| IBIS file stm32g030_031_041_tssop20.ibs
[IBIS ver] 4.2
[File name] stm32g030_031_041_tssop20.ibs
[File Rev] rev1.1
[Date]  15-05-2022
[Source] Data Created at STMicroelectronics
[Notes]  File originated from ELDO simulations.
[Disclaimer]  This information is for modeling purpose only and is
   not guaranted. The information is subject to change without
   notice.
[Copyright] Copyright 2022 STMicroelectronics Inc.
|   Component stm32g030_031_041_tssop20
[Component] stm32g030_031_041_tssop20
[Manufacturer] STMicroelectronics
[Package]
| variable   typ   min   max
R_pkg   0.0   0.0   0.0
L_pkg   0.0H   0.0H   0.0H
C_pkg   0.0F   0.0F   0.0F
[Pin]   signal_name   model_name  R_pin L_pin C_pin
1 PB8 io6_i2c_ft
2 PC14-OSCI32_IN io6_i2c_ft
3 PC15-OSC32_OUT io8prog2m25m50m120m_sudq_ft
4 VDD POWER
5 VSS GND
6 PF2-NRST io6reset
7 PA0 io6_ft
8 PA1 io6_ft
9 PA2 io6_ft
10 PA3 io6_ft
11 PA4 io6_ft
12 PA5 io6_ft
13 PA6 io6_ft
14 PA7 io6_ft
15 PB0 io6_ft
16 PA11 io6_i2c_ft
17 PA12 io6_i2c_ft
18 PA13 io6_ft
19 PA15 io6_ft
20 PB6 io6_i2c_ft
[Model Selector] io8prog2m25m50m120m_sudq_ft
iols8p_sudq_ft_pd_lv  "IO low speed, PD=40kOhm - 1P8V"
iols8p_sudq_ft_pu_lv  "IO low speed, PU=40kOhm - 1P8V"
iols8p_sudq_ft_lv  "IO low speed - 1P8V"
iols8p_sudq_ft_pd  "IO low speed, PD=40kOhm - 3P3V"
iols8p_sudq_ft_pu  "IO low speed, PU=40kOhm - 3P3V"
iols8p_sudq_ft  "IO low speed - 3P3V"
iofs8p_sudq_ft_pd_lv  "IO full speed, PD=40kOhm - 1P8V"
iofs8p_sudq_ft_pu_lv  "IO full speed, PU=40kOhm - 1P8V"
iofs8p_sudq_ft_lv  "IO full speed - 1P8V"
iofs8p_sudq_ft_pd  "IO full speed, PD=40kOhm - 3P3V"
iofs8p_sudq_ft_pu  "IO full speed, PU=40kOhm - 3P3V"
iofs8p_sudq_ft  "IO full speed - 3P3V"
ioms8p_sudq_ft_pd_lv  "IO medium speed, PD=40kOhm - 1P8V"
ioms8p_sudq_ft_pu_lv  "IO medium speed, PU=40kOhm - 1P8V"
ioms8p_sudq_ft_lv  "IO medium speed - 1P8V"
ioms8p_sudq_ft_pd  "IO medium speed, PD=40kOhm - 3P3V"
ioms8p_sudq_ft_pu  "IO medium speed, PU=40kOhm - 3P3V"
ioms8p_sudq_ft  "IO medium speed - 3P3V"
iohs8p_sudq_ft_pd_lv  "IO high speed, PD=40kOhm - 1P8V"
iohs8p_sudq_ft_pu_lv  "IO high speed, PU=40kOhm - 1P8V"
iohs8p_sudq_ft_lv  "IO high speed - 1P8V"
iohs8p_sudq_ft_pd  "IO high speed, PD=40kOhm - 3P3V"
iohs8p_sudq_ft_pu  "IO high speed, PU=40kOhm - 3P3V"
iohs8p_sudq_ft  "IO high speed - 3P3V"
[Model Selector] io6_ft
io6_ft_1v8_highspeed_pd  "GPIO-1.8V range - high speed - pull down"
io6_ft_1v8_fastspeed_pd  "GPIO-1.8V range - fast speed - pull down"
io6_ft_1v8_mediumspeed_pd  "GPIO-1.8V range - medium speed - pull down"
io6_ft_1v8_lowspeed_pd  "GPIO-1.8V range - low speed - pull down"
io6_ft_1v8_highspeed_pu  "GPIO-1.8V range - high speed - pull up"
io6_ft_1v8_fastspeed_pu  "GPIO-1.8V range - fast speed - pull up"
io6_ft_1v8_mediumspeed_pu  "GPIO-1.8V range - medium speed - pull up"
io6_ft_1v8_lowspeed_pu  "GPIO-1.8V range - low speed - pull up"
io6_ft_1v8_highspeed  "GPIO-1.8V range - high speed"
io6_ft_1v8_fastspeed  "GPIO-1.8V range - fast speed"
io6_ft_1v8_mediumspeed  "GPIO-1.8V range - medium speed"
io6_ft_1v8_lowspeed  "GPIO-1.8V range - low speed"
io6_ft_3v3_highspeed_pd  "GPIO-3.3V range - high speed - pull down"
io6_ft_3v3_fastspeed_pd  "GPIO-3.3V range - fast speed - pull down"
io6_ft_3v3_mediumspeed_pd  "GPIO-3.3V range - medium speed - pull down"
io6_ft_3v3_lowspeed_pd  "GPIO-3.3V range - low speed - pull down"
io6_ft_3v3_highspeed_pu  "GPIO-3.3V range - high speed - pull up"
io6_ft_3v3_fastspeed_pu  "GPIO-3.3V range - fast speed - pull up"
io6_ft_3v3_mediumspeed_pu  "GPIO-3.3V range - medium speed - pull up"
io6_ft_3v3_lowspeed_pu  "GPIO-3.3V range - low speed - pull up"
io6_ft_3v3_highspeed  "GPIO-3.3V range - high speed"
io6_ft_3v3_fastspeed  "GPIO-3.3V range - fast speed"
io6_ft_3v3_mediumspeed  "GPIO-3.3V range - medium speed"
io6_ft_3v3_lowspeed  "GPIO-3.3V range - low speed"
[Model Selector] io6_i2c_ft
io6_ft_1v8_highspeed_pd  "GPIO-1.8V range - high speed - pull down"
io6_ft_1v8_fastspeed_pd  "GPIO-1.8V range - fast speed - pull down"
io6_ft_1v8_mediumspeed_pd  "GPIO-1.8V range - medium speed - pull down"
io6_ft_1v8_lowspeed_pd  "GPIO-1.8V range - low speed - pull down"
io6_ft_1v8_highspeed_pu  "GPIO-1.8V range - high speed - pull up"
io6_ft_1v8_fastspeed_pu  "GPIO-1.8V range - fast speed - pull up"
io6_ft_1v8_mediumspeed_pu  "GPIO-1.8V range - medium speed - pull up"
io6_ft_1v8_lowspeed_pu  "GPIO-1.8V range - low speed - pull up"
io6_ft_1v8_highspeed  "GPIO-1.8V range - high speed"
io6_ft_1v8_fastspeed  "GPIO-1.8V range - fast speed"
io6_ft_1v8_mediumspeed  "GPIO-1.8V range - medium speed"
io6_ft_1v8_lowspeed  "GPIO-1.8V range - low speed"
io6_ft_3v3_highspeed_pd  "GPIO-3.3V range - high speed - pull down"
io6_ft_3v3_fastspeed_pd  "GPIO-3.3V range - fast speed - pull down"
io6_ft_3v3_mediumspeed_pd  "GPIO-3.3V range - medium speed - pull down"
io6_ft_3v3_lowspeed_pd  "GPIO-3.3V range - low speed - pull down"
io6_ft_3v3_highspeed_pu  "GPIO-3.3V range - high speed - pull up"
io6_ft_3v3_fastspeed_pu  "GPIO-3.3V range - fast speed - pull up"
io6_ft_3v3_mediumspeed_pu  "GPIO-3.3V range - medium speed - pull up"
io6_ft_3v3_lowspeed_pu  "GPIO-3.3V range - low speed - pull up"
io6_ft_3v3_highspeed  "GPIO-3.3V range - high speed"
io6_ft_3v3_fastspeed  "GPIO-3.3V range - fast speed"
io6_ft_3v3_mediumspeed  "GPIO-3.3V range - medium speed"
io6_ft_3v3_lowspeed  "GPIO-3.3V range - low speed"
io6_ft_1v8_highi2c_pd   "GPIO-1.8V range - high   speed i2c mode - pd"
io6_ft_1v8_fasti2c_pd   "GPIO-1.8V range - fast   speed i2c mode - pd"
io6_ft_1v8_mediumi2c_pd  "GPIO-1.8V range - medium speed i2c mode - pd"
io6_ft_1v8_lowi2c_pd   "GPIO-1.8V range - low   speed i2c mode - pd"
io6_ft_1v8_highi2c_pu   "GPIO-1.8V range - high   speed i2c mode - pu"
io6_ft_1v8_fasti2c_pu   "GPIO-1.8V range - fast   speed i2c mode - pu"
io6_ft_1v8_mediumi2c_pu  "GPIO-1.8V range - medium speed i2c mode - pu"
io6_ft_1v8_lowi2c_pu   "GPIO-1.8V range - low   speed i2c mode - pu"
io6_ft_1v8_highi2c   "GPIO-1.8V range - high   speed i2c mode"
io6_ft_1v8_fasti2c   "GPIO-1.8V range - fast   speed i2c mode"
io6_ft_1v8_mediumi2c   "GPIO-1.8V range - medium speed i2c mode"
io6_ft_1v8_lowi2c   "GPIO-1.8V range - low   speed i2c mode"
io6_ft_3v3_highi2c_pd   "GPIO-3.3V range - high   speed i2c mode - pd"
io6_ft_3v3_fasti2c_pd   "GPIO-3.3V range - fast   speed i2c mode - pd"
io6_ft_3v3_mediumi2c_pd  "GPIO-3.3V range - medium speed i2c mode - pd"
io6_ft_3v3_lowi2c_pd   "GPIO-3.3V range - low   speed i2c mode - pd"
io6_ft_3v3_highi2c_pu   "GPIO-3.3V range - high   speed i2c mode - pu"
io6_ft_3v3_fasti2c_pu   "GPIO-3.3V range - fast   speed i2c mode - pu"
io6_ft_3v3_mediumi2c_pu  "GPIO-3.3V range - medium speed i2c mode - pu"
io6_ft_3v3_lowi2c_pu   "GPIO-3.3V range - low   speed i2c mode - pu"
io6_ft_3v3_highi2c   "GPIO-3.3V range - high   speed i2c mode"
io6_ft_3v3_fasti2c   "GPIO-3.3V range - fast   speed i2c mode"
io6_ft_3v3_mediumi2c   "GPIO-3.3V range - medium speed i2c mode"
io6_ft_3v3_lowi2c   "GPIO-3.3V range - low   speed i2c mode"
io6_i2c_ft_1v8_pd  "GPIO-1.8V I2C fm+ - pd"
io6_i2c_ft_3v3_pd  "GPIO-3.3V I2C fm+ - pd"
io6_i2c_ft_1v8_pu  "GPIO-1.8V I2C fm+ - pu"
io6_i2c_ft_3v3_pu  "GPIO-3.3V I2C fm+ - pu"
io6_i2c_ft_1v8   "GPIO-1.8V I2C fm+"
io6_i2c_ft_3v3   "GPIO-3.3V I2C fm+"
[Model Selector] io6reset
io6_ft_1v8_highspeed_pd  "GPIO-1.8V range - high speed - pull down"
io6_ft_1v8_fastspeed_pd  "GPIO-1.8V range - fast speed - pull down"
io6_ft_1v8_mediumspeed_pd  "GPIO-1.8V range - medium speed - pull down"
io6_ft_1v8_lowspeed_pd  "GPIO-1.8V range - low speed - pull down"
io6_ft_1v8_highspeed_pu  "GPIO-1.8V range - high speed - pull up"
io6_ft_1v8_fastspeed_pu  "GPIO-1.8V range - fast speed - pull up"
io6_ft_1v8_mediumspeed_pu  "GPIO-1.8V range - medium speed - pull up"
io6_ft_1v8_lowspeed_pu  "GPIO-1.8V range - low speed - pull up"
io6_ft_1v8_highspeed  "GPIO-1.8V range - high speed"
io6_ft_1v8_fastspeed  "GPIO-1.8V range - fast speed"
io6_ft_1v8_mediumspeed  "GPIO-1.8V range - medium speed"
io6_ft_1v8_lowspeed  "GPIO-1.8V range - low speed"
io6_ft_3v3_highspeed_pd  "GPIO-3.3V range - high speed - pull down"
io6_ft_3v3_fastspeed_pd  "GPIO-3.3V range - fast speed - pull down"
io6_ft_3v3_mediumspeed_pd  "GPIO-3.3V range - medium speed - pull down"
io6_ft_3v3_lowspeed_pd  "GPIO-3.3V range - low speed - pull down"
io6_ft_3v3_highspeed_pu  "GPIO-3.3V range - high speed - pull up"
io6_ft_3v3_fastspeed_pu  "GPIO-3.3V range - fast speed - pull up"
io6_ft_3v3_mediumspeed_pu  "GPIO-3.3V range - medium speed - pull up"
io6_ft_3v3_lowspeed_pu  "GPIO-3.3V range - low speed - pull up"
io6_ft_3v3_highspeed  "GPIO-3.3V range - high speed"
io6_ft_3v3_fastspeed  "GPIO-3.3V range - fast speed"
io6_ft_3v3_mediumspeed  "GPIO-3.3V range - medium speed"
io6_ft_3v3_lowspeed  "GPIO-3.3V range - low speed"
ioreset_1v2_pu  "RESET 1.2V range with PU"
ioreset_1v2  "RESET 1.2V range"
ioreset_1v8_pu  "RESET 1.8V range with PU"
ioreset_1v8  "RESET 1.8V range"
ioreset_3v3_pu  "RESET 3.3V range with PU"
ioreset_3v3  "RESET 3.3V range"
| Models and submodels in the file (84): iols8p_sudq_ft_pd_lv (I/O), iols8p_sudq_ft_pu_lv (I/O), iols8p_sudq_ft_lv (I/O), iols8p_sudq_ft_pd (I/O), iols8p_sudq_ft_pu (I/O), iols8p_sudq_ft (I/O), iofs8p_sudq_ft_pd_lv (I/O), iofs8p_sudq_ft_pu_lv (I/O), iofs8p_sudq_ft_lv (I/O), iofs8p_sudq_ft_pd (I/O), iofs8p_sudq_ft_pu (I/O), iofs8p_sudq_ft (I/O), ioms8p_sudq_ft_pd_lv (I/O), ioms8p_sudq_ft_pu_lv (I/O), ioms8p_sudq_ft_lv (I/O), ioms8p_sudq_ft_pd (I/O), ioms8p_sudq_ft_pu (I/O), ioms8p_sudq_ft (I/O), iohs8p_sudq_ft_pd_lv (I/O), iohs8p_sudq_ft_pu_lv (I/O), iohs8p_sudq_ft_lv (I/O), iohs8p_sudq_ft_pd (I/O), iohs8p_sudq_ft_pu (I/O), iohs8p_sudq_ft (I/O), io6_ft_1v8_highspeed_pd (I/O), io6_ft_1v8_fastspeed_pd (I/O), io6_ft_1v8_mediumspeed_pd (I/O), io6_ft_1v8_lowspeed_pd (I/O), io6_ft_1v8_highspeed_pu (I/O), io6_ft_1v8_fastspeed_pu (I/O), io6_ft_1v8_mediumspeed_pu (I/O), io6_ft_1v8_lowspeed_pu (I/O), io6_ft_1v8_highspeed (I/O), io6_ft_1v8_fastspeed (I/O), io6_ft_1v8_mediumspeed (I/O), io6_ft_1v8_lowspeed (I/O), io6_ft_3v3_highspeed_pd (I/O), io6_ft_3v3_fastspeed_pd (I/O), io6_ft_3v3_mediumspeed_pd (I/O), io6_ft_3v3_lowspeed_pd (I/O), io6_ft_3v3_highspeed_pu (I/O), io6_ft_3v3_fastspeed_pu (I/O), io6_ft_3v3_mediumspeed_pu (I/O), io6_ft_3v3_lowspeed_pu (I/O), io6_ft_3v3_highspeed (I/O), io6_ft_3v3_fastspeed (I/O), io6_ft_3v3_mediumspeed (I/O), io6_ft_3v3_lowspeed (I/O), io6_i2c_ft_1v8_pd (I/O_open_drain), io6_i2c_ft_3v3_pd (I/O_open_drain), io6_i2c_ft_1v8_pu (I/O_open_drain), io6_i2c_ft_3v3_pu (I/O_open_drain), io6_i2c_ft_1v8 (I/O_open_drain), io6_i2c_ft_3v3 (I/O_open_drain), io6_ft_1v8_highi2c_pd (I/O_open_drain), io6_ft_1v8_fasti2c_pd (I/O_open_drain), io6_ft_1v8_mediumi2c_pd (I/O_open_drain), io6_ft_1v8_lowi2c_pd (I/O_open_drain), io6_ft_1v8_highi2c_pu (I/O_open_drain), io6_ft_1v8_fasti2c_pu (I/O_open_drain), io6_ft_1v8_mediumi2c_pu (I/O_open_drain), io6_ft_1v8_lowi2c_pu (I/O_open_drain), io6_ft_1v8_highi2c (I/O_open_drain), io6_ft_1v8_fasti2c (I/O_open_drain), io6_ft_1v8_mediumi2c (I/O_open_drain), io6_ft_1v8_lowi2c (I/O_open_drain), io6_ft_3v3_highi2c_pd (I/O_open_drain), io6_ft_3v3_fasti2c_pd (I/O_open_drain), io6_ft_3v3_mediumi2c_pd (I/O_open_drain), io6_ft_3v3_lowi2c_pd (I/O_open_drain), io6_ft_3v3_highi2c_pu (I/O_open_drain), io6_ft_3v3_fasti2c_pu (I/O_open_drain), io6_ft_3v3_mediumi2c_pu (I/O_open_drain), io6_ft_3v3_lowi2c_pu (I/O_open_drain), io6_ft_3v3_highi2c (I/O_open_drain), io6_ft_3v3_fasti2c (I/O_open_drain), io6_ft_3v3_mediumi2c (I/O_open_drain), io6_ft_3v3_lowi2c (I/O_open_drain), ioreset_1v2_pu (I/O_open_drain), ioreset_1v2 (I/O_open_drain)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
